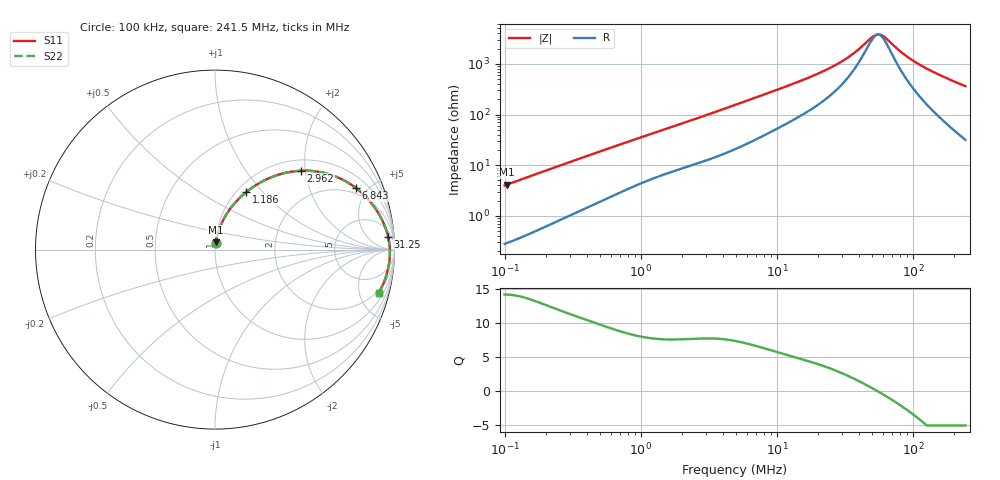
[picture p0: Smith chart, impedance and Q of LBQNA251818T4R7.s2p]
! LBQNA251818T4R7  S-PARAMETER MODEL  ( General Type )
! Model Generated by TAIYO YUDEN Corporation (http://www.ty-top.com)
! Version 1.0
! TAIYO YUDEN Control No. 191025NI43SB-FBB
! Copyright(c) 2019 TAIYO YUDEN CO.,LTD. All Rights Reserved.
! Product Description (link to TY-COMPAS)
! https://ds.yuden.co.jp/TYCOMPAS/or/detail?pn=LBQNA251818T4R7M&u=M
! Products Name : Inductors
! Characteristics :
!  Inductance : 4.7 uH , SRF(min) : 46 MHz , DC Resistance(max) : 0.169 Ohm
!  Rated Current : Saturation :340 mA , Temp Rise : 820 mA (20 degC)
!  Case Size : 2.5 x 1.8 / 0.098 x 0.071 [mm/inch] , Thickness : 1.8 / 0.071 [mm/inch]
!  (Conditions: Temperature = 25 degC , DC Bias Current/Voltage = 0A / 0V)
! External Node Assignments :
!  1  o---GGG---o  2
! GND o---------o GND
! Frequency Range : 0.1MHz  -  241.513628MHz  [ 402 STEP ]
# MHz S RI R 50
! Freq[MHz].  S11 Real  S11 Imag  S21 Real  S21 Imag  S12 Real  S12 Imag  S22 Real  S22 Imag
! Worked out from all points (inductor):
!   401 points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, 100 kHz to 241.5 MHz, reference 50 ohm
!   read as one part in series: L = 6.29 uH near 104 kHz
!   highest Q = 14.2 at 104 kHz (marker M1), where L = 6.32 uH
!   self-resonance near 55.09 MHz
!   S11 on the Smith chart (normalised r, x): 100 kHz: 1.01, +0.08; 1.186 MHz: 1.11, +0.82; 2.962 MHz: 1.24, +1.89; 6.843 MHz: 1.62, +4.20; 31.25 MHz: 10, +22; 241.5 MHz: 1.63, -7.23
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0.1  0.00435 0.0394  0.9956 -0.0394  0.9956 -0.0394  0.00435 0.0394
0.103972  0.00458 0.041  0.9954 -0.041  0.9954 -0.041  0.00458 0.041
0.368674  0.0311 0.1332  0.9689 -0.1332  0.9689 -0.1332  0.0311 0.1332
0.687508  0.0814 0.2228  0.9186 -0.2228  0.9186 -0.2228  0.0814 0.2228
1.185998  0.175 0.3212  0.825 -0.3212  0.825 -0.3212  0.175 0.3212
1.359207  0.2081 0.346  0.7919 -0.346  0.7919 -0.346  0.2081 0.346
2.961963  0.4797 0.4394  0.5203 -0.4394  0.5203 -0.4394  0.4797 0.4394
4.914404  0.6826 0.4028  0.3174 -0.4028  0.3174 -0.4028  0.6826 0.4028
6.842989  0.7863 0.3423  0.2137 -0.3423  0.2137 -0.3423  0.7863 0.3423
10.7094  0.8785 0.2495  0.1215 -0.2495  0.1215 -0.2495  0.8785 0.2495
18.11814  0.9367 0.1533  0.0633 -0.1533  0.0633 -0.1533  0.9367 0.1533
24.26464  0.9547 0.1078  0.0453 -0.1078  0.0453 -0.1078  0.9547 0.1078
31.255  0.9648 0.0723  0.0352 -0.0723  0.0352 -0.0723  0.9648 0.0723
37.24223  0.9694 0.0492  0.0306 -0.0492  0.0306 -0.0492  0.9694 0.0492
48.91461  0.9736 0.0148  0.0264 -0.0148  0.0264 -0.0148  0.9736 0.0148
52.87715  0.9742 0.00509  0.0258 -0.00509  0.0258 -0.00509  0.9742 0.00509
58.28473  0.9746 -0.00704  0.0254 0.00704  0.0254 0.00704  0.9746 -0.00704
66.79689  0.9745 -0.0242  0.0255 0.0242  0.0255 0.0242  0.9745 -0.0242
86.04029  0.9723 -0.0576  0.0277 0.0576  0.0277 0.0576  0.9723 -0.0576
110.8275  0.9669 -0.0943  0.0331 0.0943  0.0331 0.0943  0.9669 -0.0943
160.4491  0.9503 -0.1574  0.0497 0.1574  0.0497 0.1574  0.9503 -0.1574
241.5136  0.911 -0.2443  0.089 0.2443  0.089 0.2443  0.911 -0.2443
